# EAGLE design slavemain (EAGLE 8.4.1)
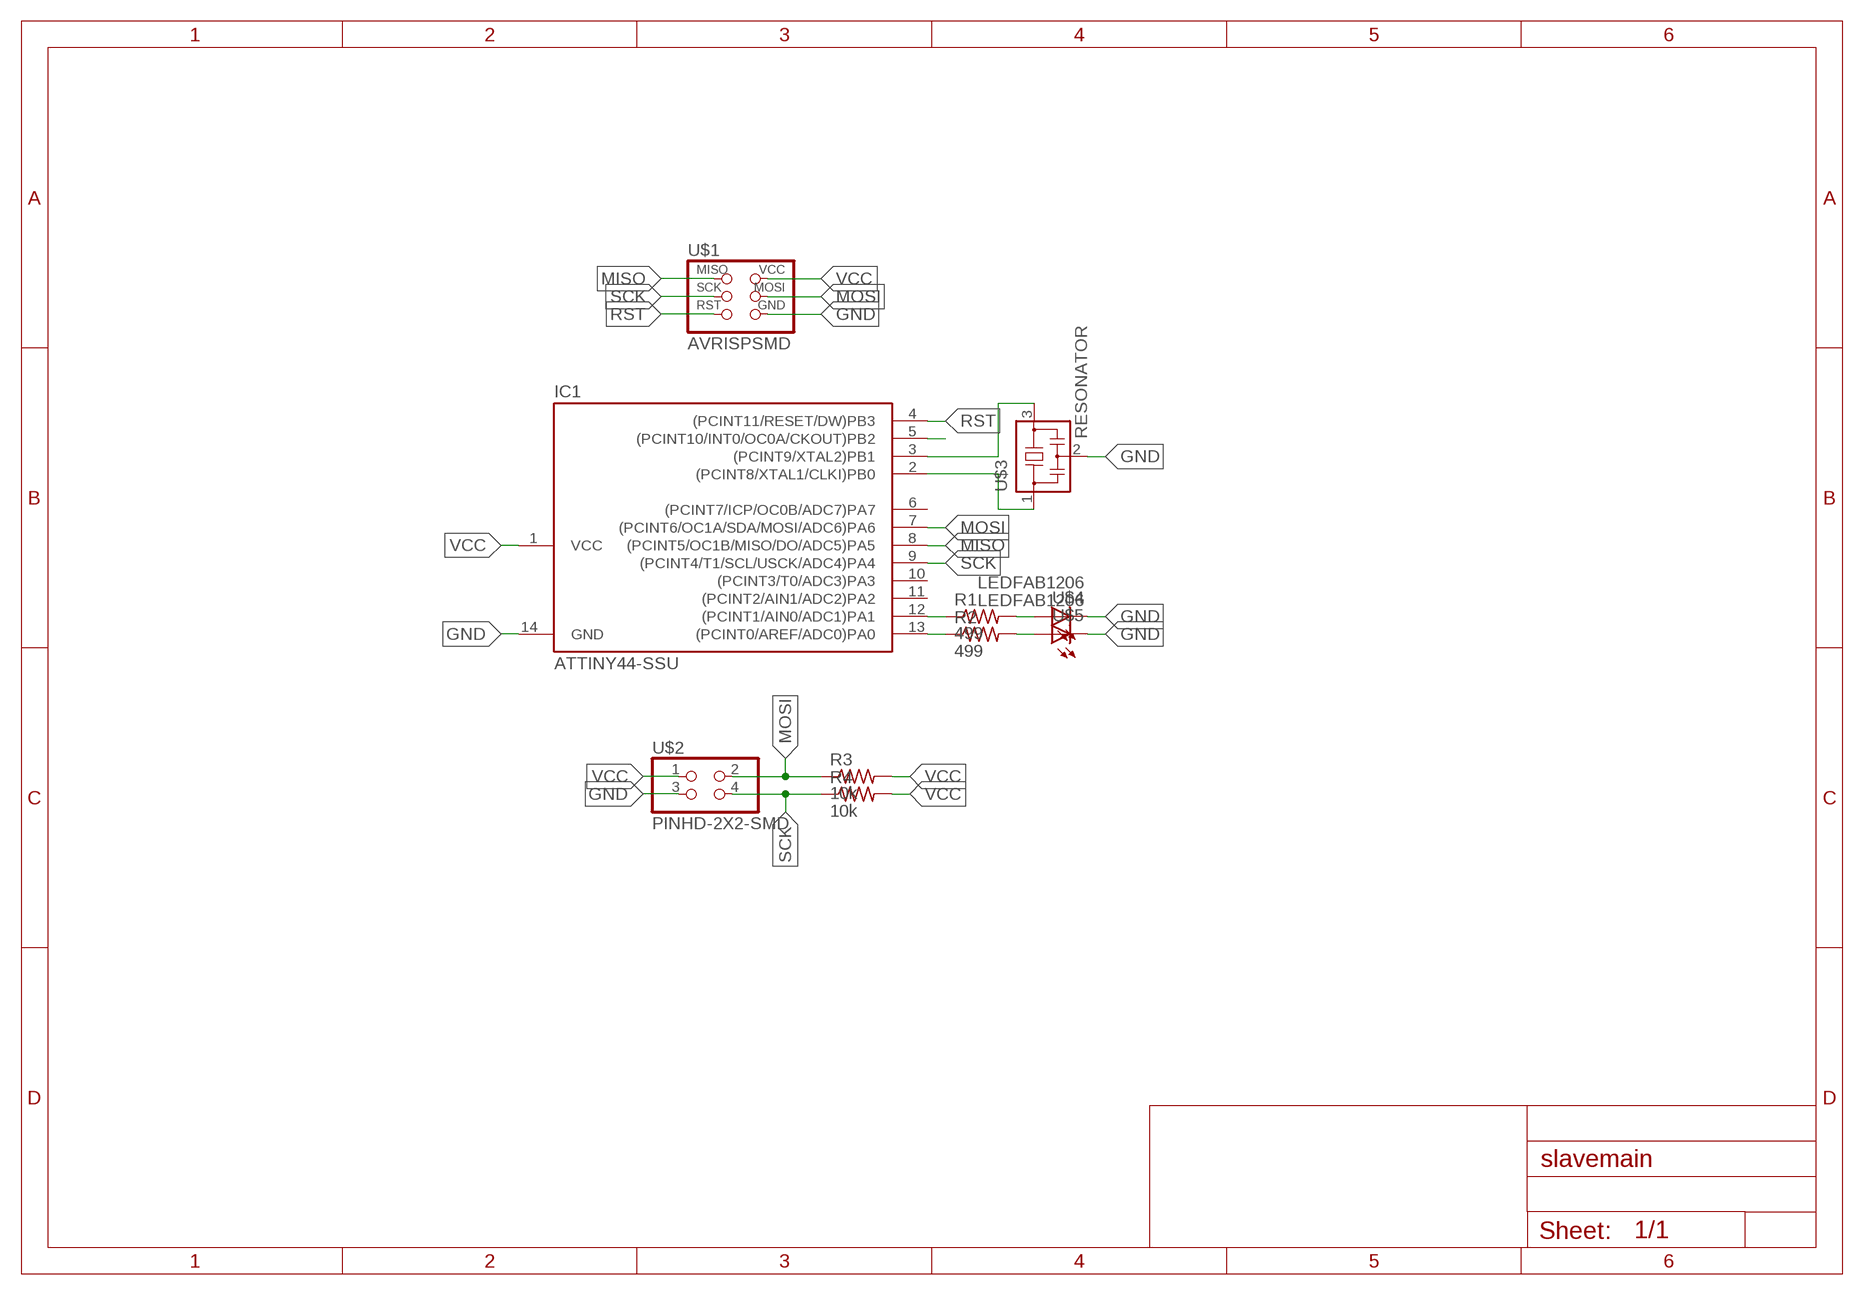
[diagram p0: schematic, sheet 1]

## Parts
IC1  ATTINY44-SSU  [SOIC14]
R1  499  RES-US1206FAB  [R1206FAB]
R2  499  RES-US1206FAB  [R1206FAB]
R3  10k  RES-US1206FAB  [R1206FAB]
R4  10k  RES-US1206FAB  [R1206FAB]
U$1  AVRISPSMD  [2X03SMD]
U$2  PINHD-2X2-SMD  [2X02SMD]
U$3  RESONATOR  [EFOBM]
U$4  LEDFAB1206  [LED1206FAB]
U$5  LEDFAB1206  [LED1206FAB]

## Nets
GND: IC1.14(GND) U$1.6(GND) U$2.3 U$3.2 U$4.2(C) U$5.2(C)
MISO: IC1.8((PCINT5/OC1B/MISO/DO/ADC5)PA5) U$1.1(MISO)
MOSI: IC1.7((PCINT6/OC1A/SDA/MOSI/ADC6)PA6) R3.1 U$1.4(MOSI) U$2.2
N$1: IC1.12((PCINT1/AIN0/ADC1)PA1) R1.1
N$2: IC1.13((PCINT0/AREF/ADC0)PA0) R2.1
N$3: R1.2 U$4.1(A)
N$4: R2.2 U$5.1(A)
N$10: IC1.5((PCINT10/INT0/OC0A/CKOUT)PB2)
N$11: IC1.3((PCINT9/XTAL2)PB1) U$3.3
N$12: IC1.2((PCINT8/XTAL1/CLKI)PB0) U$3.1
RST: IC1.4((PCINT11/RESET/DW)PB3) U$1.5(RST)
SCK: IC1.9((PCINT4/T1/SCL/USCK/ADC4)PA4) R4.1 U$1.3(SCK) U$2.4
VCC: IC1.1(VCC) R3.2 R4.2 U$1.2(VCC) U$2.1
Unconnected: IC1.6((PCINT7/ICP/OC0B/ADC7)PA7) IC1.10((PCINT3/T0/ADC3)PA3) IC1.11((PCINT2/AIN1/ADC2)PA2)

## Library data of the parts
IC1 = fab:ATTINY44
R1-R4 = fab:RES-US: Resistor (US Symbol)
U$1 = fab:AVRISP
U$2 = fab:PINHD-2X2-SMD
U$3 = fab:RESONATOR
U$4 U$5 = fab:LED: LED

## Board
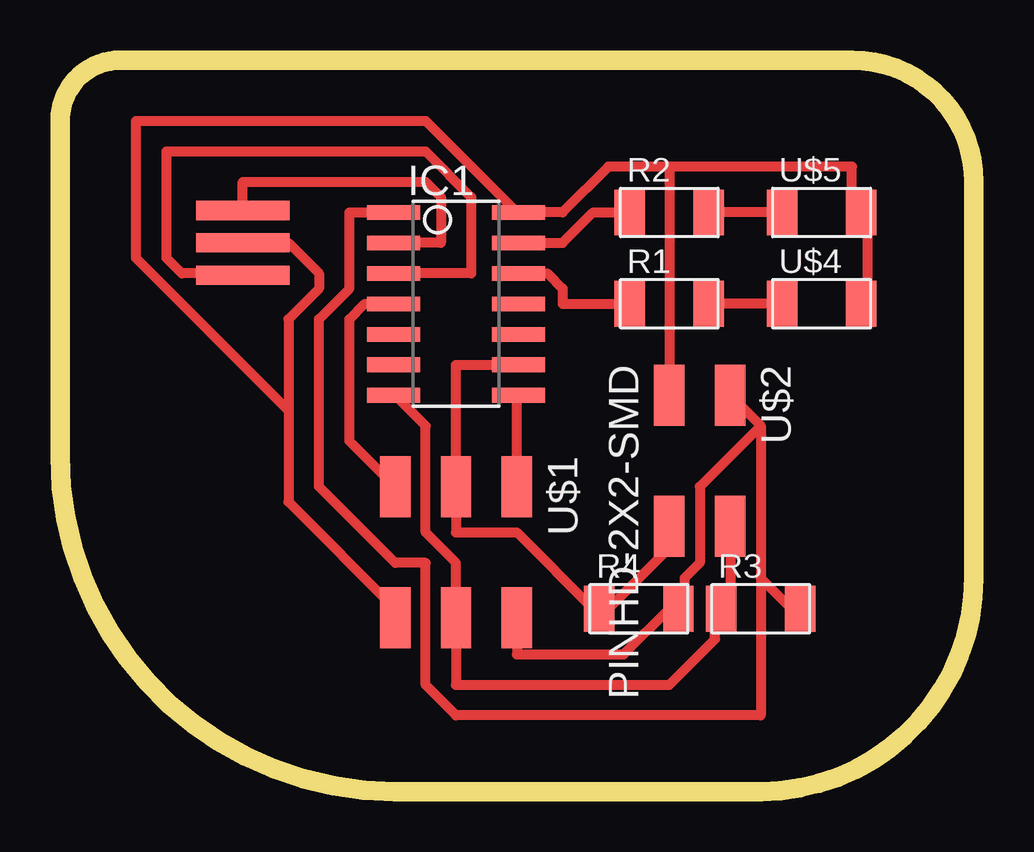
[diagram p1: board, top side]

Size 38.1 x 30.48 mm. Coordinates in mm from the lower left corner, seen from the top.
Outline: 2.54,30.48 33.02,30.48 arc-90 38.1,25.4 38.1,8.89 arc-90 29.21,0 13.97,0 arc-90 0,13.97 0,27.94 arc-90 2.54,30.48
Copper layers (1*16): Top 0.035mm / dielectric 1.5mm / Bottom 0.035mm
Design rules "default *": minimum track width 16mil, minimum drill 0.35mm, track to track 16mil, track to pad 16mil, pad to pad 16mil, via to via 16mil, smd to smd 16mil, copper to edge 16mil, drill to drill 16mil, minimum pad ring 10mil, minimum via ring 8mil, stop-mask expansion 4mil, vias tented up to drill 0mil, thermal gap 10mil

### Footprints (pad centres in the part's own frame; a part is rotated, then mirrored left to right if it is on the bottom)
SOIC14 = smd 0.61 x 2.21: 1 -3.81,-2.603; 2 -2.54,-2.603; 3 -1.27,-2.603; 4 0,-2.603; 5 1.27,-2.603; 6 2.54,-2.603; 7 3.81,-2.603; 8 3.81,2.603; 9 2.54,2.603; 10 1.27,2.603; 11 0,2.603; 12 -1.27,2.603; 13 -2.54,2.603; 14 -3.81,2.603
R1206FAB = smd 1.27 x 1.905: 1 -1.651,0; 2 1.651,0
2X03SMD = smd 2.54 x 1.27: 1 -2.54,2.54; 2 2.92,2.54; 3 -2.54,0; 4 2.92,0; 5 -2.54,-2.54; 6 2.92,-2.54
2X02SMD = smd 2.54 x 1.27: 1 -2.54,1.27; 2 2.92,1.27; 3 -2.54,-1.27; 4 2.92,-1.27
EFOBM = smd 0.8 x 3.9: 1 -1.35,0; 2 0,0; 3 1.35,0
LED1206FAB = smd 1.27 x 1.905: 1 -1.651,0; 2 1.651,0

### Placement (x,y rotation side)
IC1  16.51,20.32 270 top
R1  25.4,20.32 0 top
R2  25.4,24.13 0 top
R3  29.21,7.62 0 top
R4  24.13,7.62 0 top
U$1  16.51,10.16 270 top
U$2  26.67,13.97 270 top
U$3  7.62,22.86 270 top
U$4  31.75,20.32 0 top
U$5  31.75,24.13 0 top

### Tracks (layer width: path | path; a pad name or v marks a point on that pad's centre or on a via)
GND
  Top 0.406: U$4.2 33.66,20.32 33.66,24.13 U$5.2 33.02,24.13 33.02,26.04 25.4,26.04 | 25.4,26.04 22.86,26.04 20.96,24.13 IC1.14 19.05,24.13 15.24,27.94 3.18,27.94 3.18,22.23 9.53,15.88 | 25.4,26.04 U$2.3 | 9.53,15.88 9.53,19.69 10.79,20.96 10.79,21.59 9.53,22.86 U$3.2 | 9.53,15.88 9.53,12.07 13.97,7.62 U$1.6
MISO
  Top 0.406: U$1.1 19.05,16.51 IC1.8
MOSI
  Top 0.406: U$2.2 27.94,7.62 R3.1 27.3,7.62 27.3,6.35 25.4,4.45 16.51,4.45 U$1.4 16.51,9.52 15.24,10.8 15.24,15.24 13.97,16.51 IC1.7
N$1
  Top 0.406: R1.1 20.96,20.32 20.96,20.96 20.32,21.59 IC1.12
N$2
  Top 0.406: R2.1 22.23,24.13 20.96,22.86 IC1.13
N$3
  Top 0.406: U$4.1 R1.2
N$4
  Top 0.406: U$5.1 R2.2
N$11
  Top 0.406: IC1.3 17.14,21.59 17.14,24.77 15.24,26.67 4.45,26.67 4.45,22.23 5.08,21.59 7.62,21.59 U$3.3
N$12
  Top 0.406: IC1.2 15.87,22.86 15.87,24.77 15.24,25.4 7.62,25.4 U$3.1 7.62,24.13
RST
  Top 0.406: IC1.4 12.7,20.32 12.06,19.69 12.06,14.61 U$1.5
SCK
  Top 0.406: U$2.4 25.4,10.16 22.86,7.62 R4.1 22.23,7.62 19.05,10.8 16.51,10.8 U$1.3 16.51,17.78 IC1.9
VCC
  Top 0.406: U$1.2 19.05,5.72 23.5,5.72 25.4,7.62 R4.2 26.04,7.62 26.04,8.89 26.67,9.52 26.67,12.7 29.21,15.24 | 29.21,8.89 30.48,7.62 R3.2 | 29.21,15.24 29.21,8.89 | U$2.1 29.21,15.24 | IC1.1 12.06,24.13 12.06,20.96 10.79,19.69 10.79,12.7 13.97,9.52 15.24,9.52 15.24,4.45 16.51,3.17 29.21,3.17 29.21,8.89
